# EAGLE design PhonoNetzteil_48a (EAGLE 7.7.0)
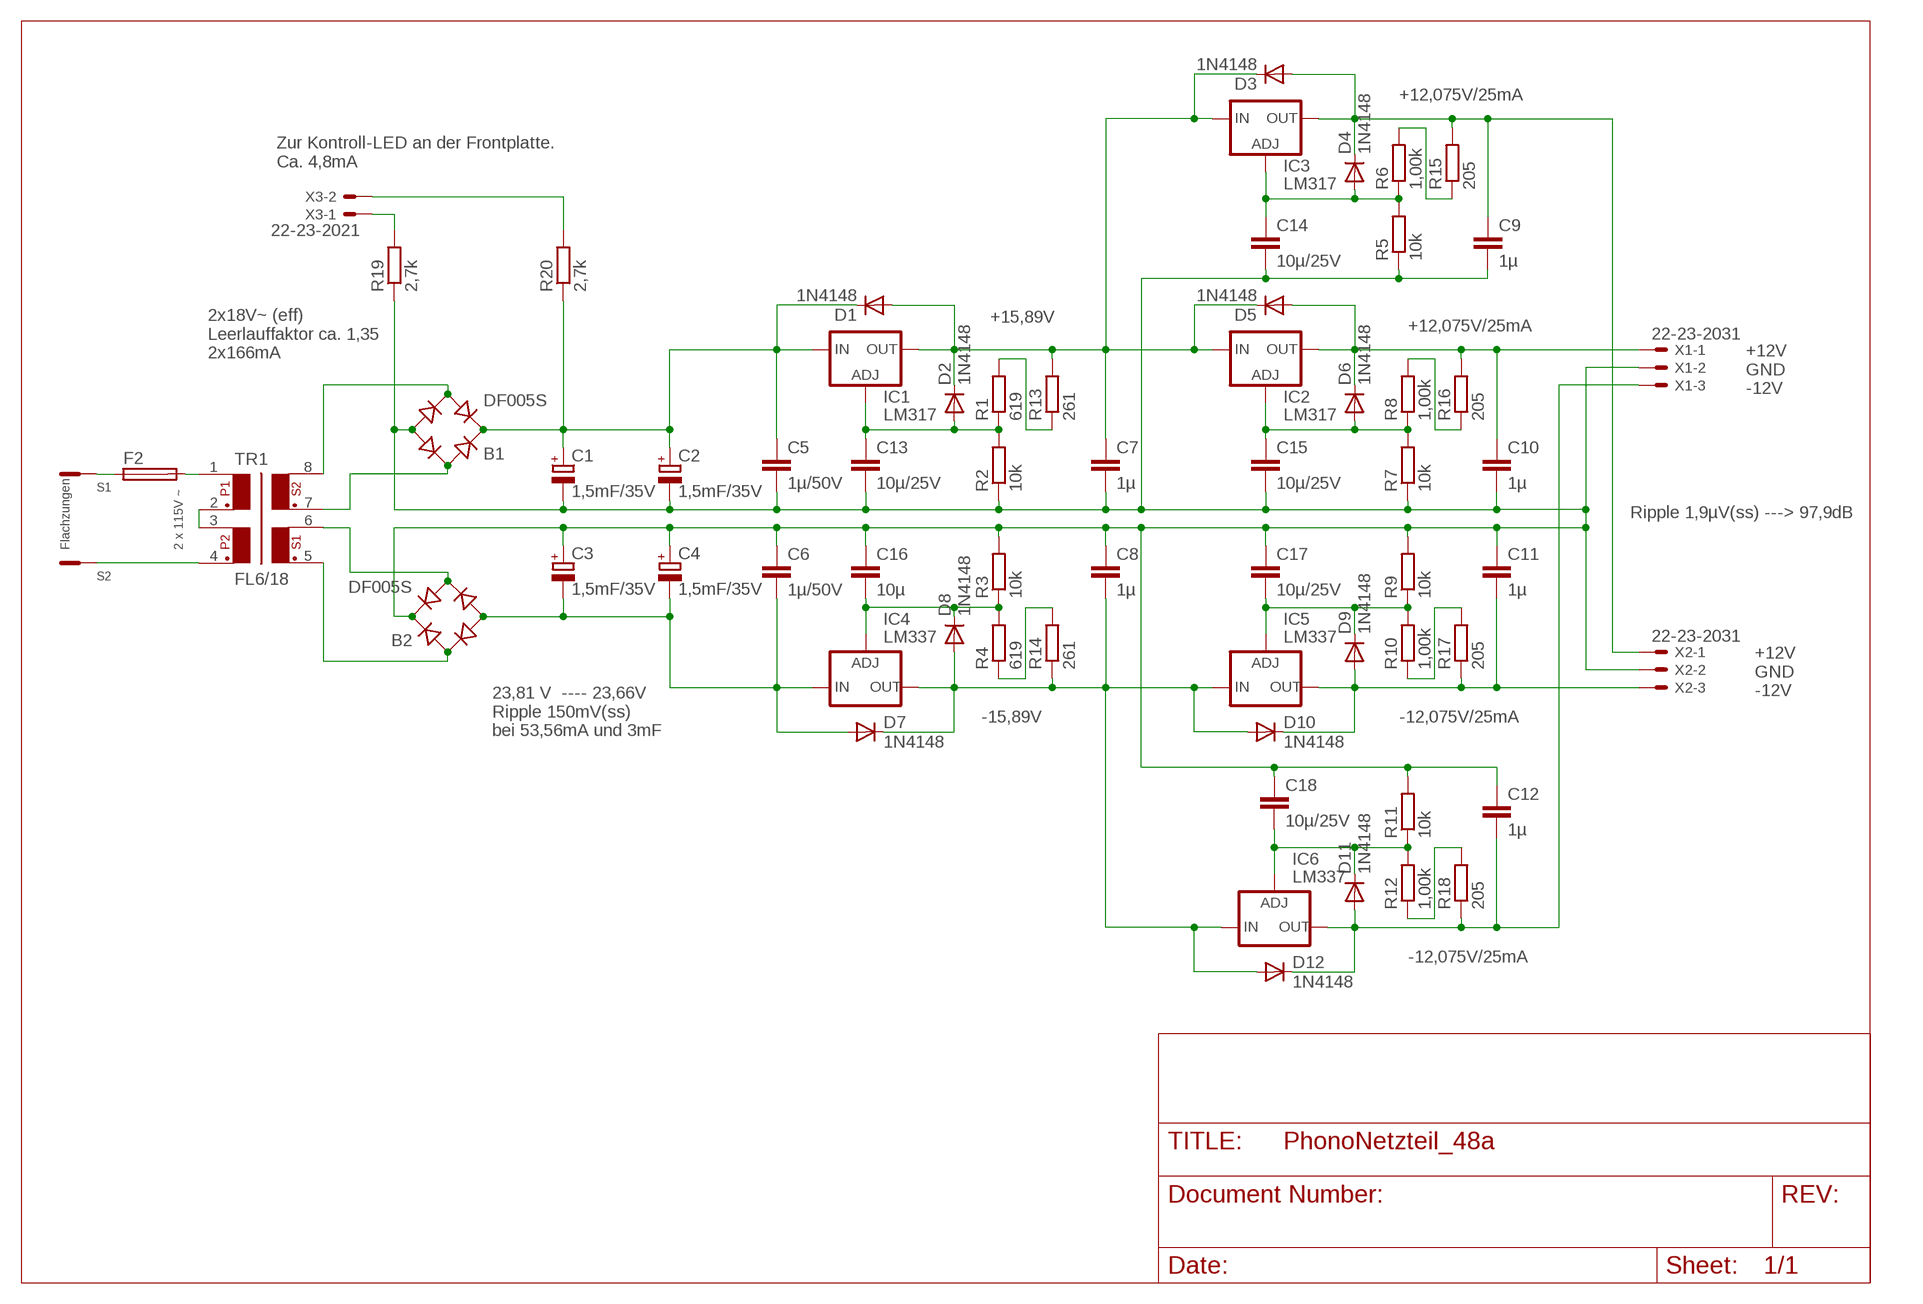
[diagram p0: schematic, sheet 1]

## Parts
B1  DF005S  [DFS]
B2  DF005S  [DFS]
C1  1,5mF/35V  CPOL-EUE7.5-18  [E7,5-18]
C2  1,5mF/35V  CPOL-EUE7.5-18  [E7,5-18]
C3  1,5mF/35V  CPOL-EUE7.5-18  [E7,5-18]
C4  1,5mF/35V  CPOL-EUE7.5-18  [E7,5-18]
C5  1µ/50V  C-EUC1206  [C1206]
C6  1µ/50V  C-EUC1206  [C1206]
C7  1µ  C-EUC1206  [C1206]
C8  1µ  C-EUC1206  [C1206]
C9  1µ  C-EUC1206  [C1206]
C10  1µ  C-EUC1206  [C1206]
C11  1µ  C-EUC1206  [C1206]
C12  1µ  C-EUC1206  [C1206]
C13  10µ/25V  C-EUC3225  [C3225]
C14  10µ/25V  C-EUC3225  [C3225]
C15  10µ/25V  C-EUC3225  [C3225]
C16  10µ  C-EUC3225  [C3225]
C17  10µ/25V  C-EUC3225  [C3225]
C18  10µ/25V  C-EUC3225  [C3225]
D1  1N4148  DIODE-SOD80C  [SOD80C]
D2  1N4148  DIODE-SOD80C  [SOD80C]
D3  1N4148  DIODE-SOD80C  [SOD80C]
D4  1N4148  DIODE-SOD80C  [SOD80C]
D5  1N4148  DIODE-SOD80C  [SOD80C]
D6  1N4148  DIODE-SOD80C  [SOD80C]
D7  1N4148  DIODE-SOD80C  [SOD80C]
D8  1N4148  DIODE-SOD80C  [SOD80C]
D9  1N4148  DIODE-SOD80C  [SOD80C]
D10  1N4148  DIODE-SOD80C  [SOD80C]
D11  1N4148  DIODE-SOD80C  [SOD80C]
D12  1N4148  DIODE-SOD80C  [SOD80C]
F2  SH22,5A  [SH22,5A]
IC1  LM317  LM317TS  [317TS]
IC2  LM317  LM317TS  [317TS]
IC3  LM317  LM317TS  [317TS]
IC4  LM337  LM337TS  [337TS]
IC5  LM337  LM337TS  [337TS]
IC6  LM337  LM337TS  [337TS]
R1  619  R-EU_R0603  [R0603]
R2  10k  R-EU_R0603  [R0603]
R3  10k  R-EU_R0603  [R0603]
R4  619  R-EU_R0603  [R0603]
R5  10k  R-EU_R0603  [R0603]
R6  1,00k  R-EU_R0603  [R0603]
R7  10k  R-EU_R0603  [R0603]
R8  1,00k  R-EU_R0603  [R0603]
R9  10k  R-EU_R0603  [R0603]
R10  1,00k  R-EU_R0603  [R0603]
R11  10k  R-EU_R0603  [R0603]
R12  1,00k  R-EU_R0603  [R0603]
R13  261  R-EU_R0603  [R0603]
R14  261  R-EU_R0603  [R0603]
R15  205  R-EU_R0603  [R0603]
R16  205  R-EU_R0603  [R0603]
R17  205  R-EU_R0603  [R0603]
R18  205  R-EU_R0603  [R0603]
R19  2,7k  R-EU_R1206  [R1206]
R20  2,7k  R-EU_R1206  [R1206]
S1  2FEET  [2FEETS]
S2  2FEET  [2FEETS]
TR1  FL6/18  FL02  [FL02-08]
X1  22-23-2031  [22-23-2031]
X2  22-23-2031  [22-23-2031]
X3  22-23-2021  [22-23-2021]

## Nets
N$1: B2.- C3.- C4.- C6.2 D7.A IC4.2(IN)
N$2: B1.+ C1.+ C2.+ C5.1 D1.C IC1.3(IN) R20.1
N$3: F2.2 TR1.1
N$4: B1.AC1 TR1.7
N$5: B1.- B2.+ C1.- C2.- C3.+ C4.+ C5.2 C6.1 C7.2 C8.1 C9.2 C10.2 C11.1 C12.1 C13.2 C14.2 C15.2 C16.1 C17.1 C18.1 R2.1 R3.2 R5.1 R7.1 R9.2 R11.2 R19.1 X1.2 X2.2
N$6: B2.AC2 TR1.6
N$7: B2.AC1 TR1.5
N$8: B1.AC2 TR1.8
N$9: C8.2 D7.C D8.A D10.A D12.A IC4.3(OUT) IC5.2(IN) IC6.2(IN) R14.1
N$10: C7.1 D1.A D2.C D3.C D5.C IC1.2(OUT) IC2.3(IN) IC3.3(IN) R13.2
N$11: R1.2 R13.1
N$12: TR1.2 TR1.3
N$13: S2.P$1 TR1.4
N$14: C13.1 D2.A IC1.1(ADJ) R1.1 R2.2
N$15: C11.2 D9.A D10.C IC5.3(OUT) R17.1 X2.3
N$16: R4.1 R14.2
N$17: C9.1 D3.A D4.C IC3.2(OUT) R15.2 X2.1
N$18: C10.1 D5.A D6.C IC2.2(OUT) R16.2 X1.1
N$19: C14.1 D4.A IC3.1(ADJ) R5.2 R6.1
N$20: C15.1 D6.A IC2.1(ADJ) R7.2 R8.1
N$21: C17.2 D9.C IC5.1(ADJ) R9.1 R10.2
N$22: C18.2 D11.C IC6.1(ADJ) R11.1 R12.2
N$23: C12.2 D11.A D12.C IC6.3(OUT) R18.1 X1.3
N$24: C16.2 D8.C IC4.1(ADJ) R3.1 R4.2
N$25: R6.2 R15.1
N$26: R8.2 R16.1
N$27: R10.1 R17.2
N$28: R12.1 R18.2
N$30: F2.1 S1.P$1
N$31: R19.2 X3.1
N$32: R20.2 X3.2

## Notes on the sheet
- +12,075V/25mA
- Zur Kontroll-LED an der Frontplatte.
  Ca. 4,8mA
- +15,89V
- +12,075V/25mA
- 2x18V~ (eff)
  Leerlauffaktor ca. 1,35
  2x166mA
- +12V
  GND
  -12V
- Ripple 1,9µV(ss) ---> 97,9dB
- Flachzungen | 2 x 115V ~
- +12V
  GND
  -12V
- -15,89V | -12,075V/25mA
- 23,81 V  ---- 23,66V
  Ripple 150mV(ss)
  bei 53,56mA und 3mF
- -12,075V/25mA

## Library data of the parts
B1 B2 = rectifier:DF*S: Surface Mount Glass Passivated Bridge Rectifiers Source: Source: Comchip Bridge Rectifiers DF005S-G thru DF10S-G.pdf
C1-C4 = rcl:CPOL-EU: POLARIZED CAPACITOR, European symbol
C5-C18 = rcl:C-EU: CAPACITOR, European symbol
D1-D12 = diode:DIODE-: DIODE
F2 = fuse:SH22,5A: FUSE HOLDER; MPN: 0031.7701.11; OC_FARNELL: unknown; OC_NEWARK: 04F1224
IC1-IC3 = v-reg:LM317TS: VOLTAGE REGULATOR
IC4-IC6 = v-reg:LM337TS: VOLTAGE REGULATOR
R1-R20 = rcl:R-EU_: RESISTOR, European symbol
S1 S2 = Steckzungen:2FEET: Steckzunge Steckbreite: 2.8 mm Steckdicke: 0.8 mm 180 ° Unisoliert Metall Vogt Verbindungstechnik 3785q08.68
TR1 = trafo:FL02: TRANSFORMER 2 primary winding, 2 secondary windings, mounting holes BLOCK
X1 X2 = con-molex:22-23-2031: .100" (2.54mm) Center Header - 3 Pin; MF: MOLEX; MPN: 22-23-2031; OC_FARNELL: 1462950; OC_NEWARK: 30C0862
X3 = con-molex:22-23-2021: .100" (2.54mm) Center Header - 2 Pin; MF: MOLEX; MPN: 22-23-2021; OC_FARNELL: 1462926; OC_NEWARK: 25C3832

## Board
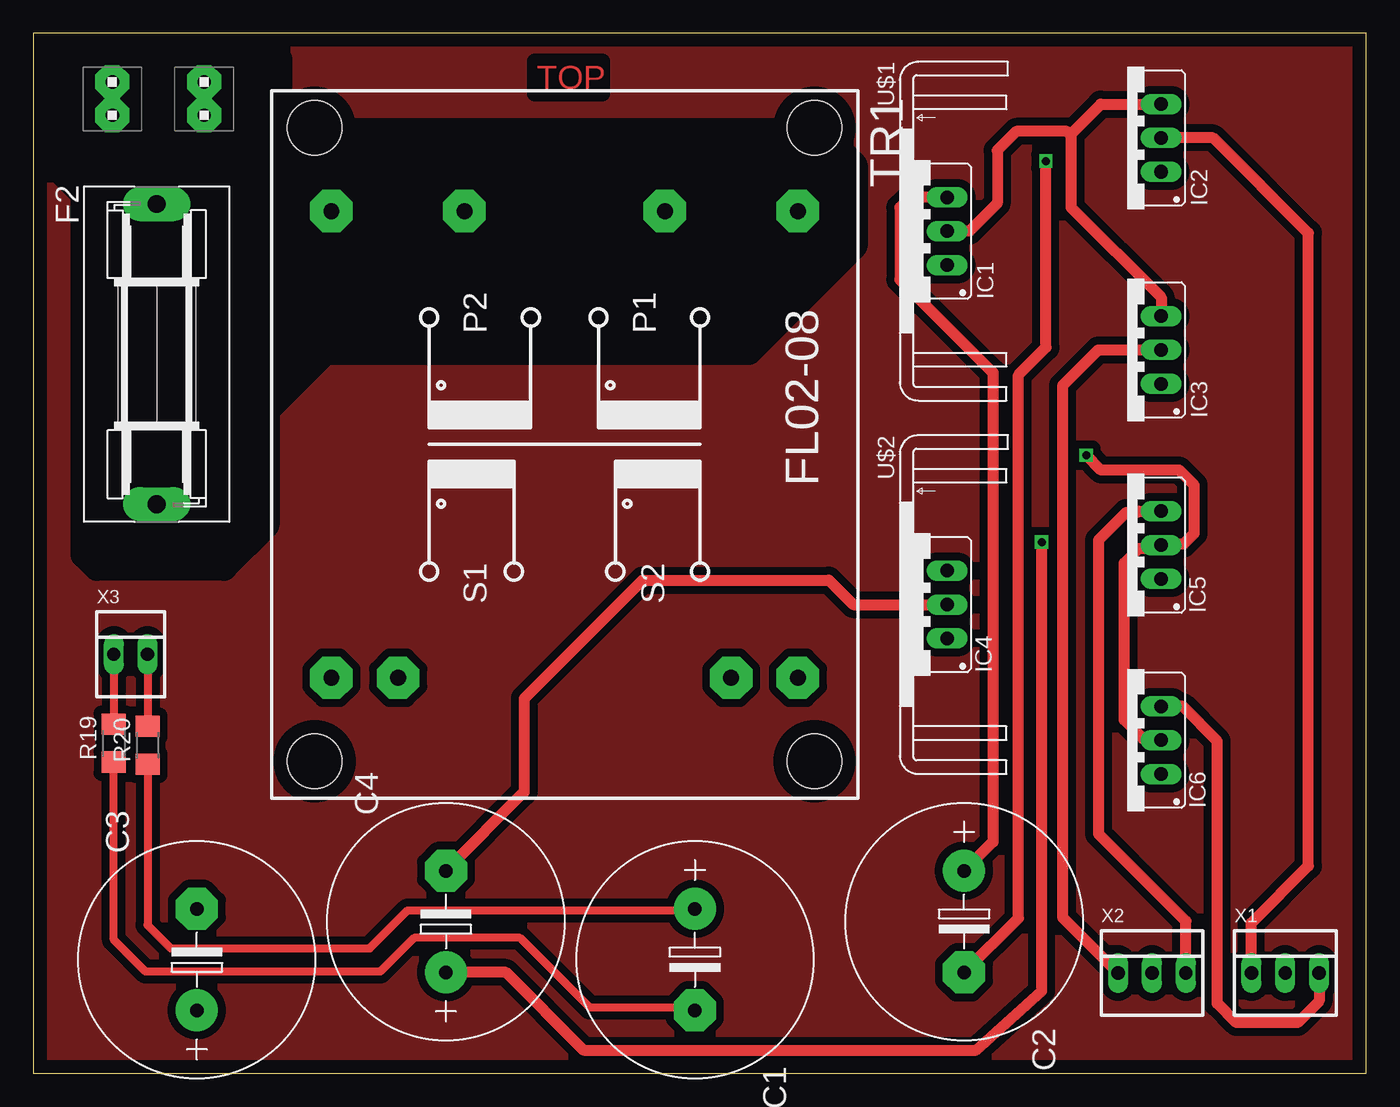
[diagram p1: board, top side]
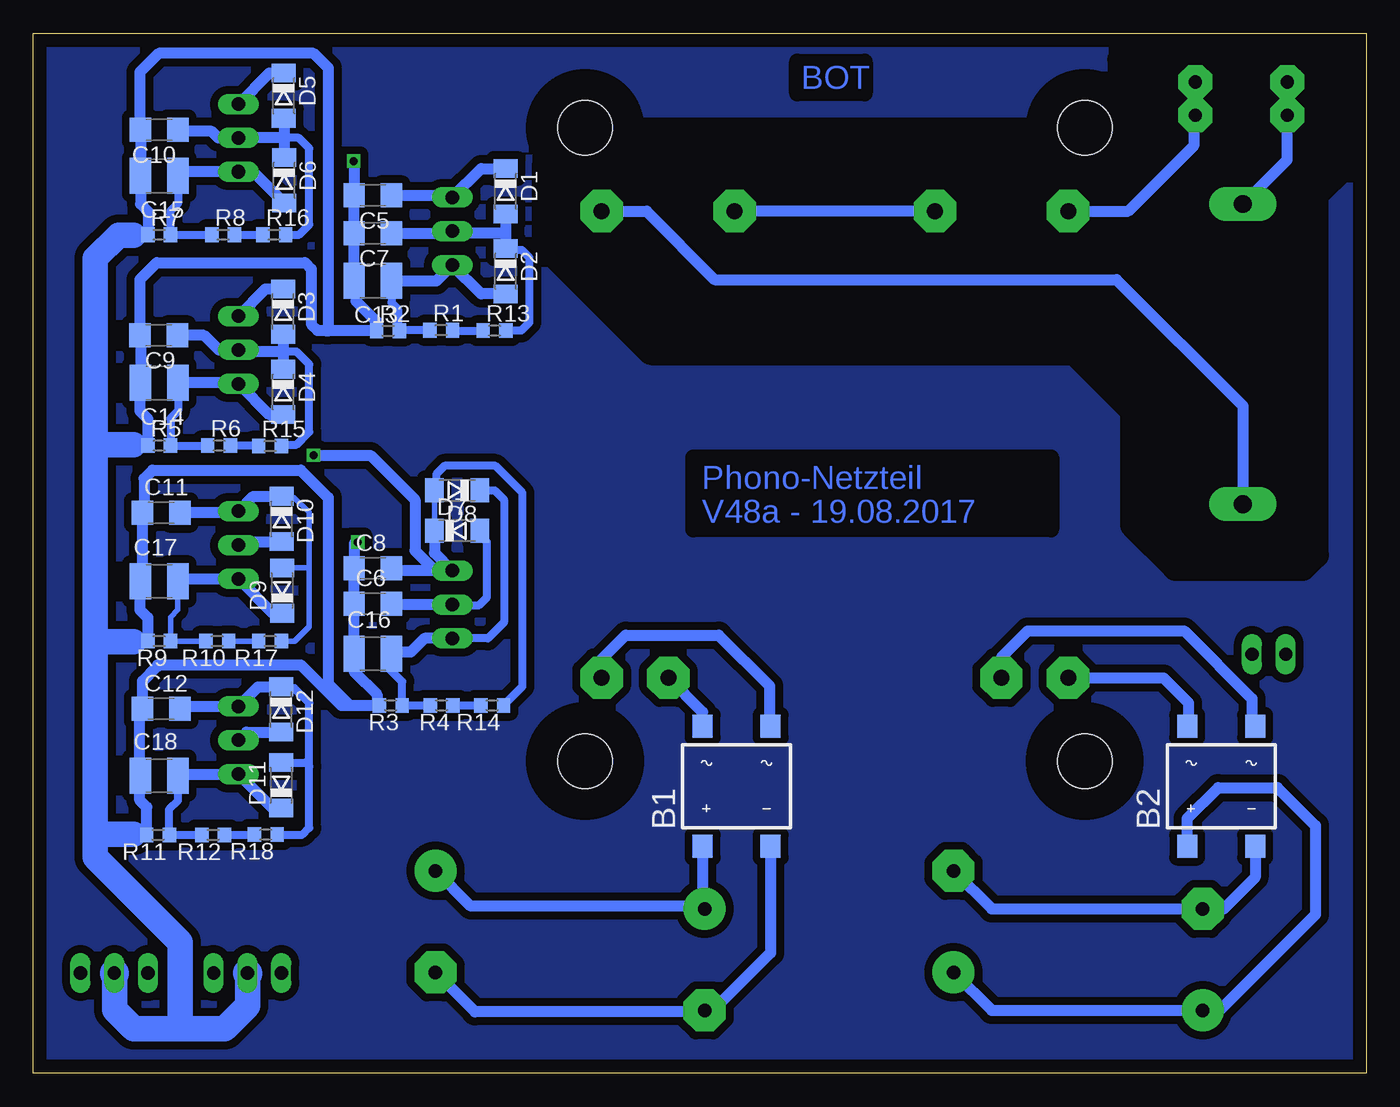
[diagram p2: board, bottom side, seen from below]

Size 100 x 78 mm. Coordinates in mm from the lower left corner, seen from the top.
Outline: 0,0 100,0 100,78 0,78 0,0
Copper layers (1*16): Top 0.035mm / dielectric 1.5mm / Bottom 0.035mm
Design rules "default": minimum track width 10mil, minimum drill 24mil, track to track 8mil, track to pad 8mil, pad to pad 8mil, via to via 8mil, smd to smd 8mil, copper to edge 40mil, drill to drill 8mil, minimum pad ring 10mil, minimum via ring 8mil, stop-mask expansion 4mil, vias tented up to drill 0mil, thermal gap 10mil
tRestrict: area 1.6,37.9 to 61.6,77.9; area 37.6,73.5 to 42.7,75.9
bRestrict: area 1.6,37.9 to 61.6,77.9; area 37.6,73.5 to 42.7,75.9; area 23.6,40.8 to 50.5,46.2

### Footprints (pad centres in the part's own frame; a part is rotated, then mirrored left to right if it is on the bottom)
DFS = smd 1.5 x 1.7: + -2.55,-4.5; - 2.55,-4.5; AC1 -2.55,4.5; AC2 2.55,4.5
E7,5-18 = drill 1.016 pad 3.15: + -3.81,0 | drill 1.016 pad 3.15 octagon: - 3.81,0
C1206 = smd 1.6 x 1.8: 1 -1.4,0; 2 1.4,0
C3225 = smd 1.6 x 2.7: 1 -1.4,0; 2 1.4,0
SOD80C = smd 1.4 x 1.8: A 1.7,0; C -1.7,0
SH22,5A = drill 1.321 pad 2.54 long: 1 -11.252,0; 2 11.252,0
317TS = drill 1.016 long: 1 -2.54,-2.54; 2 0,-2.54; 3 2.54,-2.54
337TS = drill 1.016 long: 1 -2.54,-2.54; 2 0,-2.54; 3 2.54,-2.54
R0603 = smd 1 x 1.1: 1 -0.85,0; 2 0.85,0
R1206 = smd 1.6 x 1.803: 1 -1.422,0; 2 1.422,0
2FEETS = drill 1 pad 2.54 octagon: P$1 -1.25,0; P$2 1.25,0
FL02-08 = drill 1.194 pad 3.175 octagon: 1 -17.501,17.501; 2 -17.501,7.518; 3 -17.501,-7.518; 4 -17.501,-17.501; 5 17.501,-17.501; 6 17.501,-12.497; 7 17.501,12.497; 8 17.501,17.501 | hole 4.115: 23.749,18.745; 23.749,-18.745; -23.749,-18.745; -23.749,18.745
22-23-2031 = drill 1 long: 1 -2.54,0; 2 0,0; 3 2.54,0
22-23-2021 = drill 1 long: 1 -1.27,0; 2 1.27,0

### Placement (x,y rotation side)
B1  47.23,21.53 0 bottom
B2  10.88,21.53 0 bottom
C1  49.63,8.52 270 top
C2  69.83,11.38 270 top
C3  12.27,8.52 90 top
C4  30.95,11.38 90 top
C5  74.53,65.84 180 bottom
C6  74.53,35.23 0 bottom
C7  74.53,63.01 180 bottom
C8  74.53,37.86 0 bottom
C9  90.59,55.35 180 bottom
C10  90.56,70.78 180 bottom
C11  90.41,42.06 0 bottom
C12  90.41,27.33 0 bottom
C13  74.53,59.43 180 bottom
C14  90.56,51.78 180 bottom
C15  90.56,67.3 180 bottom
C16  74.53,31.47 0 bottom
C17  90.56,36.9 0 bottom
C18  90.56,22.33 0 bottom
D1  64.56,66.16 270 bottom
D2  64.56,60.16 270 bottom
D3  81.27,57.13 270 bottom
D4  81.24,51.1 270 bottom
D5  81.21,73.33 270 bottom
D6  81.17,66.98 270 bottom
D7  68.21,40.71 0 bottom
D8  68.21,43.72 180 bottom
D9  81.34,36.21 90 bottom
D10  81.36,41.58 270 bottom
D11  81.41,21.61 90 bottom
D12  81.41,27.29 270 bottom
F2  9.26,53.94 270 top
IC1  66.03,63.16 90 top
IC2  82.07,70.16 90 top
IC3  82.07,54.25 90 top
IC4  66.03,35.16 90 top
IC5  82.07,39.62 90 top
IC6  82.07,24.98 90 top
R1  69.39,55.74 0 bottom
R2  73.39,55.69 0 bottom
R3  73.18,27.6 180 bottom
R4  69.37,27.6 180 bottom
R5  90.56,47.08 0 bottom
R6  86.07,47.08 0 bottom
R7  90.56,62.89 0 bottom
R8  85.75,62.89 0 bottom
R9  90.56,32.42 180 bottom
R10  86.19,32.42 180 bottom
R11  90.64,17.88 180 bottom
R12  86.51,17.88 180 bottom
R13  65.41,55.7 0 bottom
R14  65.57,27.6 180 bottom
R15  82.24,47.04 0 bottom
R16  81.92,62.89 0 bottom
R17  82.24,32.42 180 bottom
R18  82.56,17.91 180 bottom
R19  6.03,24.77 90 top
R20  8.57,24.61 90 top
S1  5.92,73.11 90 top
S2  12.82,73.11 90 top
TR1  39.86,47.16 270 top
U$1  [FK209]  66.03,63.16 270 top
U$2  [FK209]  66.03,35.16 270 top
X1  93.93,7.52 0 top
X2  83.93,7.52 0 top
X3  7.3,31.43 0 top

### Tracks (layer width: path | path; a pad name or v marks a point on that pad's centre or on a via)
N$1  (via drill 0.6)
  Top 0.813: v30.95,15.24 36.83,21.11 36.83,28.1 45.72,36.99 59.69,36.99 61.52,35.16 IC4.2
  Bottom 0.406: 73.22,35.16 C6.2 | IC4.2 68.49,35.08 68.51,35.08 | 66.51,40.38 D7.A
  Bottom 0.61: 68.49,35.08 66.61,35.08 65.97,35.72 65.97,39.85 66.51,40.38
  Bottom 0.813: IC4.2 73.22,35.16 | B2.- 8.33,14.69 10.69,12.33 C3.- 28.09,12.33 C4.- v30.95,15.24
N$2
  Top 0.406: 49.63,12.38 C1.+
  Top 0.61: R20.1 8.57,11.11 10.32,9.37 25.24,9.37 28.1,12.22 49.52,12.22 C1.+
  Top 0.813: IC1.3 65.79,65.7 65.02,64.93 65.02,59.53 72,52.55 72,17.36 C2.+
  Bottom 0.406: 68.71,65.84 IC1.3
  Bottom 0.813: C5.1 68.71,65.84 | IC1.3 66.41,67.86 D1.C | C1.+ 49.78,12.48 B1.+ 49.78,12.6 49.85,12.54 67.19,12.54 C2.+
N$3
  Bottom 0.813: TR1.1 53.98,64.66 53.98,64.61 48.9,59.53 18.73,59.53 9.26,50.05 F2.2
N$4
  Bottom 0.813: B1.AC1 49.78,27.09 TR1.7
N$5  (via drill 0.6)
  Top 0.406: 49.63,4.92 C1.-
  Top 0.61: 49.63,4.92 41.75,4.92 36.51,10.16 28.57,10.16 26.04,7.62 8.41,7.62 6.03,10 R19.1
  Top 0.813: v75.65,39.85 75.65,6.19 70.73,1.75 41.27,1.75 35.45,7.57 C4.+ | v75.97,68.42 75.97,54.45 73.91,52.39 73.91,11.64 C2.-
  Bottom 0.406: 75.81,57.94 75.81,59.32 | 75.81,59.32 C13.2 | 75.81,59.32 75.55,59.32 75.48,59.38 | C16.1 75.93,30.12 | 74.22,27.79 R3.2 | 92,22.38 C18.1 92,22.28 | 92,27.13 C12.1 | 92,36.86 C17.1 91.81,37.05 | 91.37,62.81 R7.1 | C9.2 91.96,55.32 | C14.2 92,51.73
  Bottom 0.61: 92.48,62.87 92.45,62.89 R7.1 | 92.48,47.15 92.41,47.08 R5.1 | 92.48,32.38 92.45,32.42 R9.2 | 95.34,16.19 95.02,16.51 95.02,17.94 | 92.48,17.94 92.42,17.88 R11.2
  Bottom 0.813: C16.1 C6.1 C8.1 75.93,39.73 75.81,39.85 v75.65,39.85 | 75.81,57.94 74.24,56.37 R2.1 77.88,55.69 | C13.2 C7.2 C5.2 75.93,68.38 v75.97,68.42 | 75.93,30.12 74.22,28.42 74.22,27.79 | 92,22.38 92,27.13 | R11.2 91.49,19.96 92,20.48 92,22.28 | 92,36.86 92,34.77 91.41,34.17 R9.2 | 91.81,37.05 C11.1 91.69,42.18 91.69,44.61 91.05,45.24 79.94,45.24 77.88,43.18 77.88,29.21 76.26,27.6 | 91.37,62.81 91.37,64.61 91.96,65.2 C15.2 C10.2 92,70.83 92,75.09 90.59,76.5 78.97,76.5 77.88,75.41 77.88,55.69 | 91.96,55.32 C14.2 | 92,51.73 92,49.69 91.41,49.09 R5.1 | C9.2 91.99,57.3 92,57.31 92,59.53 90.73,60.8 79.62,60.8 79.15,60.33 79.15,56.2 78.67,55.72 78.03,55.72 78,55.69 77.88,55.69 | 76.26,27.6 R3.2 | C12.1 91.81,29.41 90.73,30.48 arc90 90.58,30.64 79.94,30.64 76.9,27.6 76.26,27.6 | B2.+ 13.43,19.12 11.11,21.43 6.67,21.43 3.81,18.57 3.81,11.9 11,4.71 C3.+ 28.09,4.71 C4.+ | 49,4.71 C1.- | B1.- 44.69,9.03 49,4.71 | 49,4.71 49.11,4.6 66.87,4.6 C2.-
  Bottom 1.93: 92.48,62.87 93.59,62.87 95.34,61.12 95.34,16.19 88.99,9.84 88.99,3.33 | 92.48,47.15 95.02,47.15 | 94.86,32.38 92.48,32.38 | 95.02,17.94 92.48,17.94 | 83.91,7.5 83.91,5.08 85.66,3.33 88.99,3.33 | 93.91,7.5 93.91,4.76 92.48,3.33 88.99,3.33
  Bottom 2.184: X2.2 83.91,7.5 | X1.2 93.91,7.5
N$6
  Bottom 0.813: TR1.6 27.36,31.22 25.4,33.18 13.65,33.18 8.57,28.1 8.57,26.28 B2.AC2
N$7
  Bottom 0.813: TR1.5 15.22,29.66 13.34,27.78 13.34,26.12 B2.AC1
N$8
  Bottom 0.813: TR1.8 57.36,31.06 55.56,32.86 48.58,32.86 44.77,29.05 44.77,26.11 B1.AC2
N$9  (via drill 0.6)
  Top 0.254: 84.41,25.13 IC6.2
  Top 0.813: 84.41,25.13 84.37,25.08 83.27,25.08 81.84,26.51 81.84,38.26 82.96,39.37 84.36,39.37 IC5.2 84.68,39.69 86.29,39.69 87.08,40.48 87.08,44.13 85.97,45.24 80.1,45.24 v78.99,46.35
  Bottom 0.406: D7.C D8.A 69.78,43.84 | 72.96,37.7 C8.2
  Bottom 0.61: 69.78,43.84 69.78,44.93 69.14,45.56 65.33,45.56 63.3,43.53 63.3,29.02 R14.1
  Bottom 0.813: IC4.3 72.96,37.7 | D7.C 69.91,39.04 IC4.3 | IC5.2 84.36,39.88 D10.A | IC6.2 84.01,25.59 D12.A | v78.99,46.35 74.7,46.35 71.37,43.02 71.37,39.21 69.86,37.7 IC4.3
N$10  (via drill 0.6)
  Top 0.813: IC2.3 80.09,72.7 77.88,70.48 77.88,70.33 | IC3.3 84.61,58.19 77.88,64.93 77.88,70.33 | 77.88,70.33 77.56,70.64 73.75,70.64 72.32,69.22 72.32,65.25 70.23,63.16 IC1.2
  Bottom 0.406: 64.56,63.16 64.7,63.02 | 68.43,63.02 IC1.2 68.72,63.01 C7.1 | 64.46,61.75 D2.C
  Bottom 0.61: 64.46,61.75 63.35,61.75 62.8,61.2 62.8,56.3 63.4,55.7 R13.2
  Bottom 0.813: D2.C D1.A 64.56,63.16 | 64.7,63.02 68.43,63.02 | IC3.3 82.57,58.83 D3.C | IC2.3 82.28,75.03 D5.C | C7.1 68.51,63.01 v68.51,63.18
N$11
  Bottom 0.406: R1.2 68.51,55.7
  Bottom 0.61: 68.51,55.7 R13.1
N$12
  Bottom 0.813: TR1.3 TR1.2
N$13
  Bottom 0.813: TR1.4 17.86,64.66 12.9,69.62 12.9,71.78 S2.P$1
N$14
  Bottom 0.406: R1.1 72.49,55.74 R2.2 72.64,55.79 | 72.46,55.74 72.48,55.72
  Bottom 0.61: R1.1 72.46,55.74 | C13.1 73.13,57.8 72.64,57.31 72.64,55.79
  Bottom 0.813: D2.A 66.41,58.46 IC1.1 69.75,59.43 C13.1
N$15
  Top 0.813: X2.3 86.47,11.41 79.94,17.94 79.94,40.01 82,42.07 82.8,42.07 82.89,42.16 IC5.3
  Bottom 0.406: IC5.3 84.72,42.06 | R17.1 80.38,32.42 79.31,33.5 79.31,37.94 | 79.31,37.94 79.31,42.07 80.42,43.18 81.27,43.18 D10.C | D9.A 79.33,37.91 79.31,37.94
  Bottom 0.813: 84.72,42.06 C11.2 | IC5.3 83.5,43.28 D10.C
N$16
  Bottom 0.61: R4.1 R14.2
N$17
  Top 0.813: IC3.2 79.9,54.25 77.24,51.59 77.24,11.67 X2.1
  Bottom 0.406: 81.27,52.83 D4.C | R15.2 81.28,47.15 | 83.75,54.13 83.87,54.25
  Bottom 0.61: 81.28,47.15 80.26,47.15 79.31,48.1 79.31,53.18 80.26,54.13 81.27,54.13
  Bottom 0.813: D3.A 81.27,54.13 | 81.27,54.13 81.27,52.83 | C9.1 87.19,55.35 86.09,54.25 IC3.2 83.87,54.25 | 81.27,54.13 83.75,54.13
N$18
  Top 0.813: IC2.2 88.52,70.16 95.66,63.02 95.66,15.56 91.37,11.27 91.37,7.54 X1.1
  Bottom 0.406: D5.A 81.17,71.91 | 89.02,70.64 C10.1 | D6.C 81.21,68.71 81.21,70.16 | 81.04,62.87 R16.2
  Bottom 0.61: 81.21,70.16 80.09,70.16 79.31,69.37 79.31,63.66 80.1,62.87 81.04,62.87
  Bottom 0.813: 81.17,71.91 D6.C | 89.02,70.64 86.61,70.64 86.12,70.16 IC2.2 81.21,70.16
N$19
  Bottom 0.406: IC3.1 84.68,51.78 | C14.1 89.15,51.77
  Bottom 0.61: R6.1 R5.2 89.71,49.13 89.15,49.69 89.15,51.77
  Bottom 0.813: 84.68,51.78 C14.1 | IC3.1 82.3,49.4 D4.A
N$20
  Bottom 0.406: 88.84,67.62 C15.1 89.15,67.29
  Bottom 0.61: R8.1 R7.2 89.71,64.68 89.15,65.25 89.15,67.29
  Bottom 0.813: 88.84,67.62 IC2.1 83.52,67.62 D6.A
N$21
  Bottom 0.406: R10.2 R9.1 | R9.1 89.47,32.43 | 88.98,37.08 C17.2 89.16,34.75 89.71,34.2 R9.1
  Bottom 0.813: 88.98,37.08 IC5.1 82.05,34.51 D9.C
N$22
  Bottom 0.406: 89.15,22.32 C18.2 89.05,22.44 | D11.C 81.63,19.68 81.85,19.68
  Bottom 0.61: 89.15,22.32 89.15,20.48 89.79,19.84 R11.1 R12.2
  Bottom 0.813: 89.05,22.44 IC6.1 81.85,19.68
N$23
  Top 0.813: X1.3 96.47,5.42 94.86,3.81 90.26,3.81 88.83,5.24 88.83,24.92 86.23,27.52 IC6.3
  Bottom 0.406: C12.2 88.81,27.52 | 79.59,23.31 79.31,23.02
  Bottom 0.61: R18.1 79.81,17.91 79.31,18.41 79.31,23.02 79.31,27.78 80.42,28.89 81.31,28.89 D12.C | D11.A 79.59,23.31
  Bottom 0.813: 88.81,27.52 IC6.3 83.15,28.99 D12.C
N$24
  Bottom 0.406: 68.49,32.54 IC4.1 | 73.27,30.32 73.27,31.32 C16.2 73.01,31.59
  Bottom 0.61: 73.27,30.32 72.33,29.38 R3.1 R4.2 | IC4.1 65.89,32.62 64.7,33.81 64.7,43.02 65.39,43.72 D8.C
  Bottom 0.813: IC4.1 70.66,32.62 71.69,31.59 73.01,31.59
N$25
  Bottom 0.406: R15.1 83.13,47.08
  Bottom 0.61: 83.13,47.08 R6.2
N$26
  Bottom 0.61: R8.2 R16.1
N$27
  Bottom 0.406: R17.2 R10.1
N$28
  Bottom 0.406: 83.44,17.88 R18.2
  Bottom 0.61: R12.1 83.44,17.88
N$29
  pour Bottom (isolate 0.6): 0,0 0,78 100,78 100,0
  pour Top (isolate 0.6): 0.32,-0.32 0.32,78 100.32,78 100.32,-0.32
N$30
  Bottom 0.813: F2.1 5.92,68.52 S1.P$1
N$31
  Top 0.61: X3.1 R19.2
N$32
  Top 0.61: 8.57,26.35 R20.2 X3.2

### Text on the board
Top: TOP
Bottom: BOT | Phono-Netzteil | V48a - 19.08.2017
